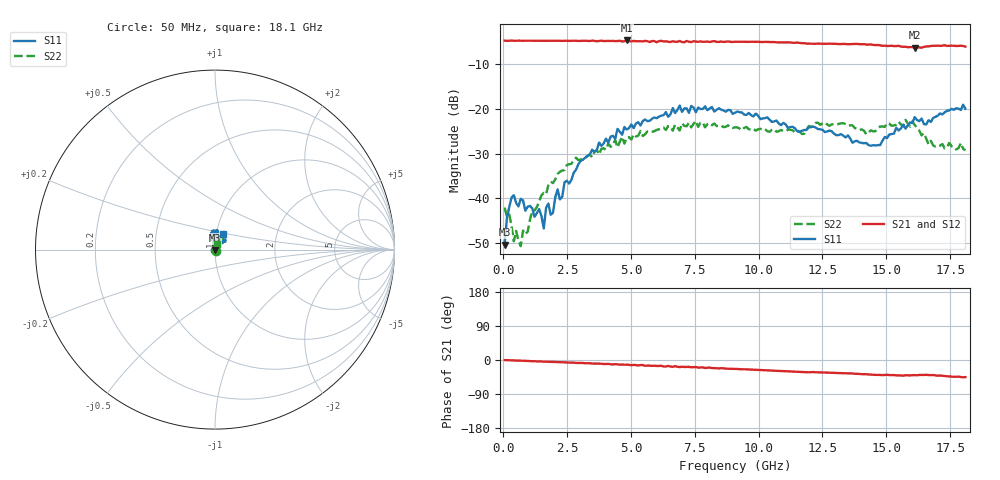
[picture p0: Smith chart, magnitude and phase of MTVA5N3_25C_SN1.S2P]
! Network Analyzer HP8720D.06.14 Serial No. US36140669
! 11 May 2005  11:24:25
! Frequency  S11  S21  S12  S22
# HZ  S  DB R 50
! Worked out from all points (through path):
!   201 points, 50 MHz to 18.1 GHz, reference 50 ohm
!   highest |S21| = -4.70 dB at 4.833 GHz (marker M1); lowest = -6.3 dB at 16.11 GHz (marker M2)
!   group delay of S21, straight-line fit = 7.04 ps
!   lowest |S11| = -50.4 dB at 50 MHz (marker M3), VSWR 1.01, Z = 50 - j0.302 ohm
!   |S11| at or under -10 dB: start of sweep to end of sweep
!   |S22| runs from -50.7 to -22.5 dB; largest |S21 - S12| = 0.021
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5e7  -50.39 -86.9  -4.75 -0.2  -4.76 -0.7  -42.09 -58.2
1.4025e8  -44.48 -148.0  -4.80 -0.4  -4.81 -0.9  -44.13 -13.0
3.2075e8  -39.85 -171.0  -4.73 -0.8  -4.75 -1.1  -46.21 -32.4
4.11e8  -39.32 -166.3  -4.76 -1.2  -4.77 -1.6  -49.65 9.7
6.8175e8  -40.12 177.0  -4.75 -1.8  -4.76 -2.3  -50.73 41.2
1.40375e9  -42.44 150.7  -4.76 -3.7  -4.77 -4.1  -40.74 89.2
1.58425e9  -46.77 125.8  -4.77 -4.2  -4.78 -4.6  -38.81 83.6
1.76475e9  -41.21 125.0  -4.78 -4.7  -4.76 -5.0  -37.09 86.9
1.94525e9  -43.24 91.7  -4.78 -5.0  -4.78 -5.5  -36.62 84.4
2.12575e9  -38.02 96.4  -4.76 -5.6  -4.77 -5.9  -34.58 86.5
2.30625e9  -39.70 75.3  -4.79 -6.0  -4.78 -6.3  -33.80 87.6
2.3965e9  -36.44 76.6  -4.78 -6.2  -4.78 -6.6  -33.70 90.2
3.1185e9  -31.39 74.1  -4.78 -7.9  -4.80 -8.5  -31.27 112.2
4.83325e9  -24.64 81.8  -4.70 -12.3  -4.78 -13.4  -26.44 87.8
6.09675e9  -21.75 82.7  -4.85 -15.8  -4.80 -16.2  -24.58 83.4
9.075e9  -20.86 99.9  -4.98 -23.6  -4.95 -24.0  -24.14 67.7
1.21435e10  -23.97 103.8  -5.43 -31.8  -5.40 -32.4  -23.85 73.2
1.439975e10  -28.25 52.8  -5.59 -38.5  -5.57 -38.8  -24.80 72.5
1.512175e10  -25.73 48.2  -5.92 -39.8  -5.81 -39.9  -23.33 74.8
1.61145e10  -21.85 44.2  -6.33 -39.9  -6.14 -40.7  -23.62 61.5
1.6656e10  -22.55 55.1  -6.04 -39.8  -5.95 -39.5  -27.94 53.3
1.81e10  -19.99 63.2  -6.08 -45.2  -6.08 -46.5  -29.26 73.5
